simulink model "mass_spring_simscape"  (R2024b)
settings: Solver=VariableStepAuto  StartTime=0.0  StopTime=20  RelTol=1e-3
libraries: fl_lib x6, nesl_utility x3

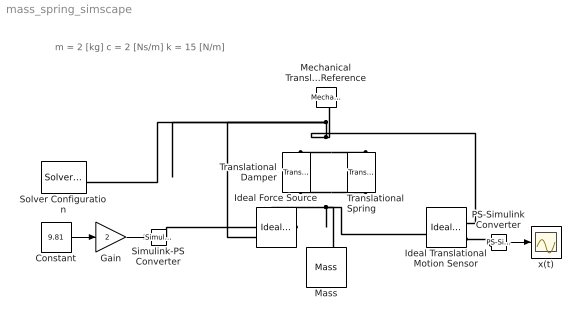
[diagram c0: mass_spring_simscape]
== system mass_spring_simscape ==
  note: m = 2 [kg] c = 2 [Ns/m] k = 15 [N/m]
  Constant : Constant  Value=9.81
  Gain : Gain  Gain=2
  Ideal Force Source : fl_lib/Mechanical/Mechanical Sources/Ideal Force Source
  Ideal Translational Motion Sensor : fl_lib/Mechanical/Mechanical Sensors/Ideal Translational Motion Sensor  reference=foundation.enum.MeasurementReference.difference  acceleration_port=false  velocity_port=true  position_port=true  offset=0 m
  Mass : fl_lib/Mechanical/Translational Elements/Mass  mass=2 kg  num_ports=foundation.enum.numPorts2.one  v_specify=off  v_priority=High  v=0 m/s  v_nominal_specify=off  v_nominal_value=1  v_nominal_unit=m/s  f_specify=off  f_priority=None  f=0 N  f_nominal_specify=off  f_nominal_value=1  f_nominal_unit=N
  Mechanical Translational Reference : fl_lib/Mechanical/Translational Elements/Mechanical Translational Reference
  PS-Simulink Converter : nesl_utility/PS-Simulink Converter  PhysicalDomain=network_engine_domain  SubClassName=ps_output  LeftPortType=input  RightPortType=output  PseudoPeriodic=off  Frequencies=[]  VectorFormat=inherit  Unit=inherit  AffineConversion=off
  Simulink-PS Converter : nesl_utility/Simulink-PS Converter  PhysicalDomain=network_engine_domain  SubClassName=ps_input  LeftPortType=input  RightPortType=output  PseudoPeriodic=off  Frequencies=[]  NoiseDistribution=none  NoiseParameters=[]  Unit=1  AffineConversion=off  FilteringAndDerivatives=provide  SimscapeFilterOrder=1  InputFilterTimeConstant=0.001  UdotUserProvided=0
  Solver Configuration : nesl_utility/Solver Configuration  PhysicalDomain=network_engine_domain  SubClassName=solver  LeftPortType=input  RightPortType=generic  Tones=[]  Harmonics=[]  SimulateNoise=off  Profile=off  UseLocalSampling=off  EnableSwitchedLinearOptims=on  FrequencyDomain=off  UseCCode=off  RelTol=0.001  AbsTol=0.001  MinStep=1e-09  ToWorkspace=off  RevertToSquareIcSolve=off  NumHomotopyIterations=100  PhasorMode=off  PhasorModeNumHarmonics=1  ConsistencySolver=NEWTON_XTOL_AFTER_FTOL  IndexReductionMethod=DerivativeReplacement  DoDC=off  ResidualTolerance=1e-09  ConsistencyTolSource=GLOBAL  ConsistencyAbsTol=0.001  ConsistencyRelTol=0.001  ConsistencyTolFactor=0.001  UseLocalSolver=off  LocalSolverChoice=NE_BACKWARD_EULER_ADVANCER  ResolveIndetEquations=on  FunctionEvalNumThread=1  LocalSolverSampleTime=0.001  DoFixedCost=off  MaxNonlinIter=3  MaxModeIter=2  ComputeImpulses=off  ImpulseIterations=2  LinearAlgebra=auto  LinearAlgebraNumThread=0  EquationFormulation=NE_TIME_EF  DelaysMemoryBudget=1024  AutomaticFiltering=on  FilteringTimeConstant=0.001  PartitionStorageMethod=AS_NEEDED  PartitionMemoryBudget=1024  PartitionMethod=ROBUST  MultibodyUseLocalSolver=off  MultibodyLocalSolverChoice=ODE1  MultibodyLocalSolverSampleTime=0.001
  Translational Damper : fl_lib/Mechanical/Translational Elements/Translational Damper  D=2 N*s/m  v_specify=off  v_priority=None  v=0 m/s  v_nominal_specify=off  v_nominal_value=1  v_nominal_unit=m/s  f_specify=off  f_priority=None  f=0 N  f_nominal_specify=off  f_nominal_value=1  f_nominal_unit=N
  Translational Spring : fl_lib/Mechanical/Translational Elements/Translational Spring  spr_rate=15 N/m  v_specify=off  v_priority=None  v=0 m/s  v_nominal_specify=off  v_nominal_value=1  v_nominal_unit=m/s  f_specify=off  f_priority=None  f=0 N  f_nominal_specify=off  f_nominal_value=1  f_nominal_unit=N  x_specify=off  x_priority=High  x=0 m  x_nominal_specify=off  x_nominal_value=1  x_nominal_unit=m
  x(t) : Scope
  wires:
  Constant/1 -> Gain/1
  Gain/1 -> Simulink-PS Converter/1
  PS-Simulink Converter/1 -> x(t)/1
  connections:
  Translational Damper/RConn1 -- Solver Configuration/RConn1 -- Ideal Force Source/RConn2 -- Mechanical Translational Reference/LConn1 -- Ideal Translational Motion Sensor/RConn1 -- Translational Spring/RConn1
  Translational Damper/LConn1 -- Mass/LConn1 -- Ideal Translational Motion Sensor/LConn1 -- Ideal Force Source/LConn1 -- Translational Spring/LConn1
  Simulink-PS Converter/RConn1 -- Ideal Force Source/RConn1
  PS-Simulink Converter/LConn1 -- Ideal Translational Motion Sensor/RConn3
